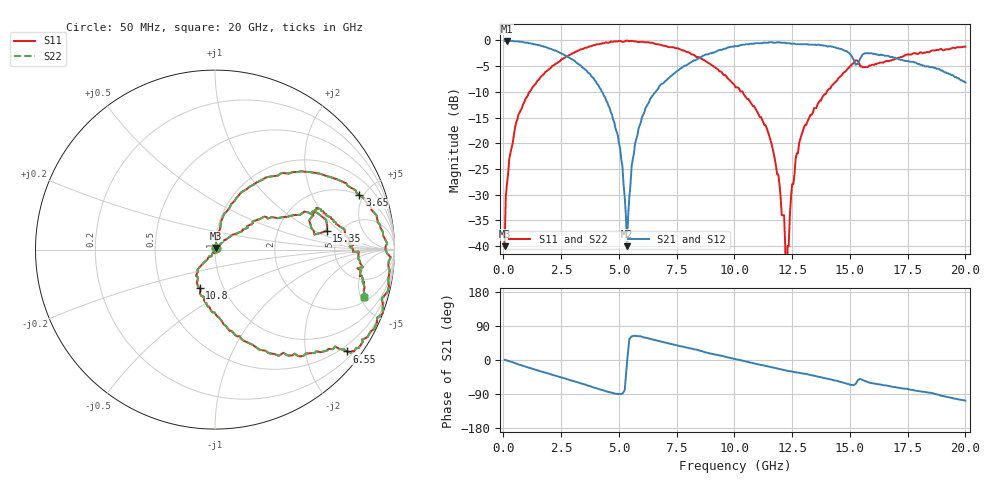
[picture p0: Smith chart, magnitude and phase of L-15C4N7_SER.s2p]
# MHZ S MA R 50
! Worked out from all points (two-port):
!   400 points, 50 MHz to 20 GHz, reference 50 ohm
!   highest |S21| = -0.09 dB at 150 MHz (marker M1); lowest = -40.0 dB at 5.35 GHz (marker M2)
!   |S21| within 3 dB of the highest: start of sweep to 2.746 GHz; 8.604 GHz to 15.08 GHz (6.477 GHz wide, 54.7 % of centre)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
!   lowest |S11| = -40.0 dB at 50 MHz (marker M3), VSWR 1.02, Z = 50.3 + j0.956 ohm
!   |S11| at or under -10 dB: start of sweep to 1.131 GHz; 10.36 GHz to 13.99 GHz (3.632 GHz wide, 29.8 % of centre)
!   |S22| runs from - to 0.0 dB; largest |S21 - S12| = 0
!   S11 on the Smith chart (normalised r, x): 50 MHz: 1.01, +0.02; 3.65 GHz: 2.01, +4.67; 6.55 GHz: 0.35, -2.90; 10.8 GHz: 0.77, -0.35; 15.35 GHz: 3.91, +1.35; 20 GHz: 2.43, -5.31
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50  0.01 71.8  0.99 0.7  0.99 0.7  0.01 71.8
150  0.04 83.2  0.99 -1.3  0.99 -1.3  0.04 83.2
950  0.27 70.4  0.95 -17.3  0.95 -17.3  0.27 70.4
3400  0.82 25.7  0.55 -62.6  0.55 -62.6  0.82 25.7
3650  0.86 20.6  0.49 -67.5  0.49 -67.5  0.86 20.6
4950  0.98 -10.0  0.12 -89.3  0.12 -89.3  0.98 -10.0
5350  1 -20.8  0.01 -6.7  0.01 -6.7  1 -20.8
5700  0.98 -28.8  0.1 63.7  0.1 63.7  0.98 -28.8
6550  0.93 -37.6  0.31 52.5  0.31 52.5  0.93 -37.6
6700  0.92 -37.9  0.34 50.5  0.34 50.5  0.92 -37.9
10050  0.35 -90.4  0.88 2.3  0.88 2.3  0.35 -90.4
10800  0.23 -111.7  0.93 -8.1  0.93 -8.1  0.23 -111.7
11550  0.11 -130.8  0.96 -18.5  0.96 -18.5  0.11 -130.8
12150  0.02 -94.6  0.95 -26.8  0.95 -26.8  0.02 -94.6
12200  0.01 -65.7  0.95 -27.5  0.95 -27.5  0.01 -65.7
12250  0 -36.8  0.94 -28.3  0.94 -28.3  0 -36.8
12300  0.01 -13.7  0.94 -28.8  0.94 -28.8  0.01 -13.7
12450  0.03 47.1  0.93 -30.0  0.93 -30.0  0.03 47.1
13350  0.19 36.0  0.91 -40.2  0.91 -40.2  0.19 36.0
15350  0.63 9.5  0.59 -53.1  0.59 -53.1  0.63 9.5
16700  0.63 20.0  0.7 -69.0  0.7 -69.0  0.63 20.0
20000  0.87 -17.8  0.39 -107.1  0.39 -107.1  0.87 -17.8
